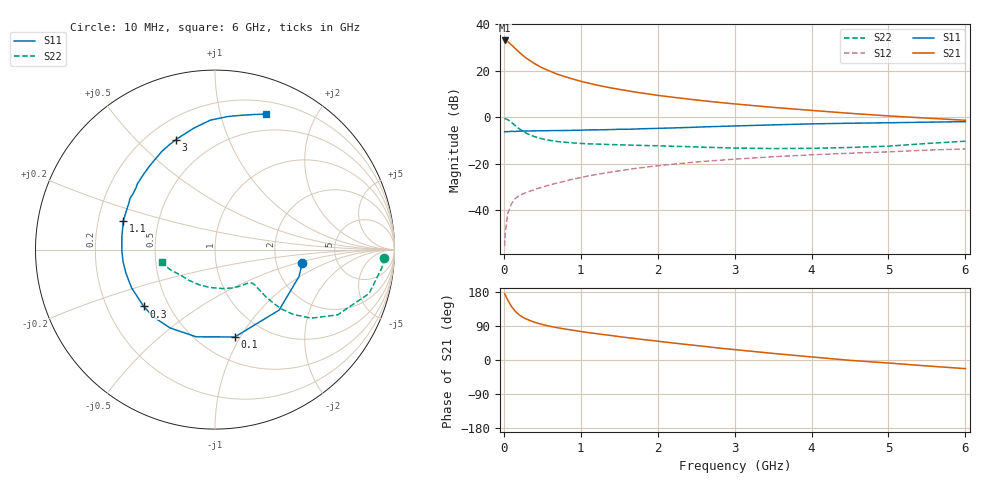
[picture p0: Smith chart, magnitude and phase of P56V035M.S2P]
! SIEMENS Small Signal Semiconductors
! BFP183
! Si NPN RF Bipolar Junction Transistor in SOT143
! VCE = 6 V  IC = 35 mA
! Common Emitter S-Parameters:  March  1996
# GHz  S  MA  R  50
!  f  S11  S21  S12  S22
! GHz  MAG  ANG  MAG  ANG  MAG  ANG  MAG  ANG
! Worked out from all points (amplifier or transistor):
!   36 points, 10 MHz to 6 GHz, reference 50 ohm
!   highest |S21| = 33.0 dB at 10 MHz (marker M1)
!   |S21| within 3 dB of that: start of sweep to 133.9 MHz
!   unconditionally stable (mu >= 1): 663.2 MHz to 5.725 GHz
!   at 250 MHz: K = 0.58, MSG = 29.7 dB, |S12| = -32.9 dB
!   at 1.4 GHz: K = 1.16, MAG = 15.6 dB, |S12| = -23.5 dB
!   at 6 GHz: K = 0.97, MSG = 6.2 dB, |S12| = -13.6 dB
!   S11 on the Smith chart (normalised r, x): 10 MHz: 2.81, -0.56; 100 MHz: 0.73, -0.95; 300 MHz: 0.36, -0.31; 1.1 GHz: 0.31, +0.14; 3 GHz: 0.31, +0.66; 6 GHz: 0.32, +1.40
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0.01  0.4917 -8.8  44.77 175.0  0.0017 80.3  0.9441 -2.8
0.02  0.4915 -17.8  44.68 171.1  0.0034 86.7  0.9344 -6.4
0.05  0.4911 -43.3  42.34 158.3  0.0085 77.4  0.8928 -15.9
0.1  0.4992 -77.2  35.85 141.1  0.0139 62.5  0.7741 -28.0
0.15  0.4971 -102.2  29.91 128.2  0.0181 55.9  0.658 -35.5
0.2  0.5032 -119.8  24.98 119.1  0.0208 52.8  0.567 -39.6
0.25  0.5076 -132.2  21.13 112.4  0.0227 52.0  0.4996 -41.7
0.3  0.5081 -141.4  18.28 107.4  0.0246 50.8  0.4477 -42.5
0.4  0.5113 -155.4  14.23 99.4  0.028 52.5  0.3824 -42.8
0.5  0.5134 -165.2  11.54 93.7  0.0317 53.1  0.343 -42.4
0.6  0.5167 -172.4  9.786 89.0  0.0353 54.6  0.318 -42.0
0.7  0.5188 -178.9  8.379 85.0  0.0391 55.5  0.3011 -41.6
0.8  0.5201 175.9  7.411 81.5  0.0425 56.3  0.2899 -41.7
1  0.5284 166.6  5.943 75.2  0.0505 57.1  0.2745 -42.6
1.1  0.5355 162.5  5.432 72.3  0.0551 57.2  0.2692 -43.4
1.5  0.5528 149.0  3.98 61.6  0.0708 55.7  0.2561 -48.2
2.2  0.5905 128.4  2.693 44.9  0.0982 50.5  0.2382 -61.7
3  0.6506 109.6  1.939 27.4  0.1261 42.9  0.2179 -82.3
3.5  0.6871 99.9  1.633 17.4  0.1417 38.3  0.2129 -97.5
4.5  0.7449 84.5  1.218 -0.9  0.1691 28.8  0.2247 -130.5
5.5  0.7839 73.8  0.96 -15.7  0.1973 20.9  0.2736 -155.8
6  0.8069 69.3  0.863 -22.8  0.2094 16.2  0.3061 -166.6
